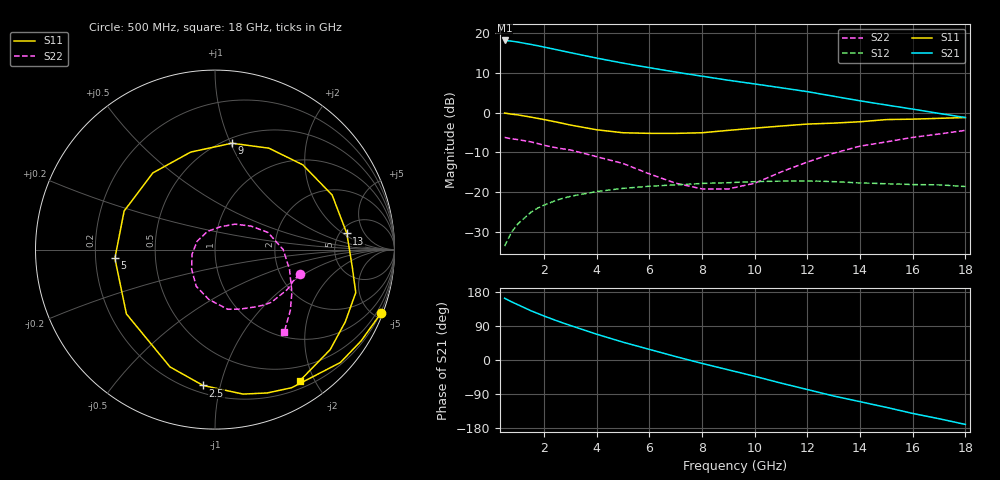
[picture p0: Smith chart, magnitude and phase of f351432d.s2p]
!ATF-35143
!S-PARAMETERS at Vds=2V  Id=30mA.  LAST UPDATED 06-3-99
# ghz s ma r 50
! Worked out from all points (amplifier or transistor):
!   23 points, 500 MHz to 18 GHz, reference 50 ohm
!   highest |S21| = 18.2 dB at 500 MHz (marker M1)
!   |S21| within 3 dB of that: start of sweep to 2.952 GHz
!   unconditionally stable (mu >= 1): 7.131 GHz to end of sweep
!   at 1.5 GHz: K = 0.31, MSG = 21.1 dB, |S12| = -25.0 dB
!   at 7 GHz: K = 0.99, MSG = 14.2 dB, |S12| = -18.1 dB
!   at 18 GHz: K = 1.27, MAG = 5.6 dB, |S12| = -18.6 dB
!   lowest NFmin = 0.11 dB at 500 MHz
!   S11 on the Smith chart (normalised r, x): 500 MHz: 0.15, -5.39; 2.5 GHz: 0.25, -0.89; 5 GHz: 0.28, -0.04; 9 GHz: 0.55, +1.01; 13 GHz: 5.75, +2.29; 18 GHz: 0.30, -1.80
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0.5  0.99 -21.0  8.1 163.0  0.021 77.0  0.49 -16.0
0.75  0.96 -32.0  7.96 154.0  0.031 71.0  0.47 -22.0
1  0.94 -42.0  7.73 146.0  0.04 65.0  0.46 -29.0
1.5  0.88 -61.0  7.22 130.0  0.056 55.0  0.43 -43.0
1.75  0.85 -70.0  6.96 123.0  0.063 50.0  0.41 -49.0
2  0.82 -79.0  6.69 116.0  0.069 46.0  0.39 -55.0
2.5  0.76 -95.0  6.17 103.0  0.08 37.0  0.36 -67.0
3  0.7 -111.0  5.69 91.0  0.089 29.0  0.34 -78.0
4  0.61 -144.0  4.86 68.0  0.102 15.0  0.28 -97.0
5  0.56 -175.0  4.2 47.0  0.112 2.0  0.23 -117.0
6  0.55 157.0  3.68 28.0  0.119 -11.0  0.17 -140.0
7  0.55 129.0  3.24 9.0  0.124 -24.0  0.13 -169.0
8  0.56 104.0  2.88 -9.0  0.129 -35.0  0.11 155.0
9  0.6 81.0  2.56 -26.0  0.132 -46.0  0.11 112.0
10  0.64 62.0  2.3 -43.0  0.136 -57.0  0.13 77.0
11  0.68 44.0  2.06 -61.0  0.138 -69.0  0.18 52.0
12  0.72 25.0  1.84 -78.0  0.139 -81.0  0.24 33.0
13  0.74 7.0  1.61 -95.0  0.136 -93.0  0.31 18.0
14  0.77 -7.0  1.41 -110.0  0.131 -103.0  0.38 0.0
15  0.82 -17.0  1.25 -125.0  0.128 -113.0  0.43 -15.0
16  0.83 -29.0  1.11 -141.0  0.125 -124.0  0.49 -29.0
18  0.87 -57.0  0.87 -170.0  0.118 -145.0  0.6 -50.0
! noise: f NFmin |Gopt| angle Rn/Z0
0.5  0.11  0.87  3  0.18
0.9  0.15  0.81  12  0.17
1.5  0.22  0.73  26  0.15
1.8  0.25  0.69  33  0.15
2.5  0.33  0.6  51  0.13
3  0.39  0.54  64  0.12
5  0.64  0.39  127  0.07
6  0.77  0.34  161  0.05
8  1.02  0.33  -130  0.1
10  1.28  0.4  -67  0.3
